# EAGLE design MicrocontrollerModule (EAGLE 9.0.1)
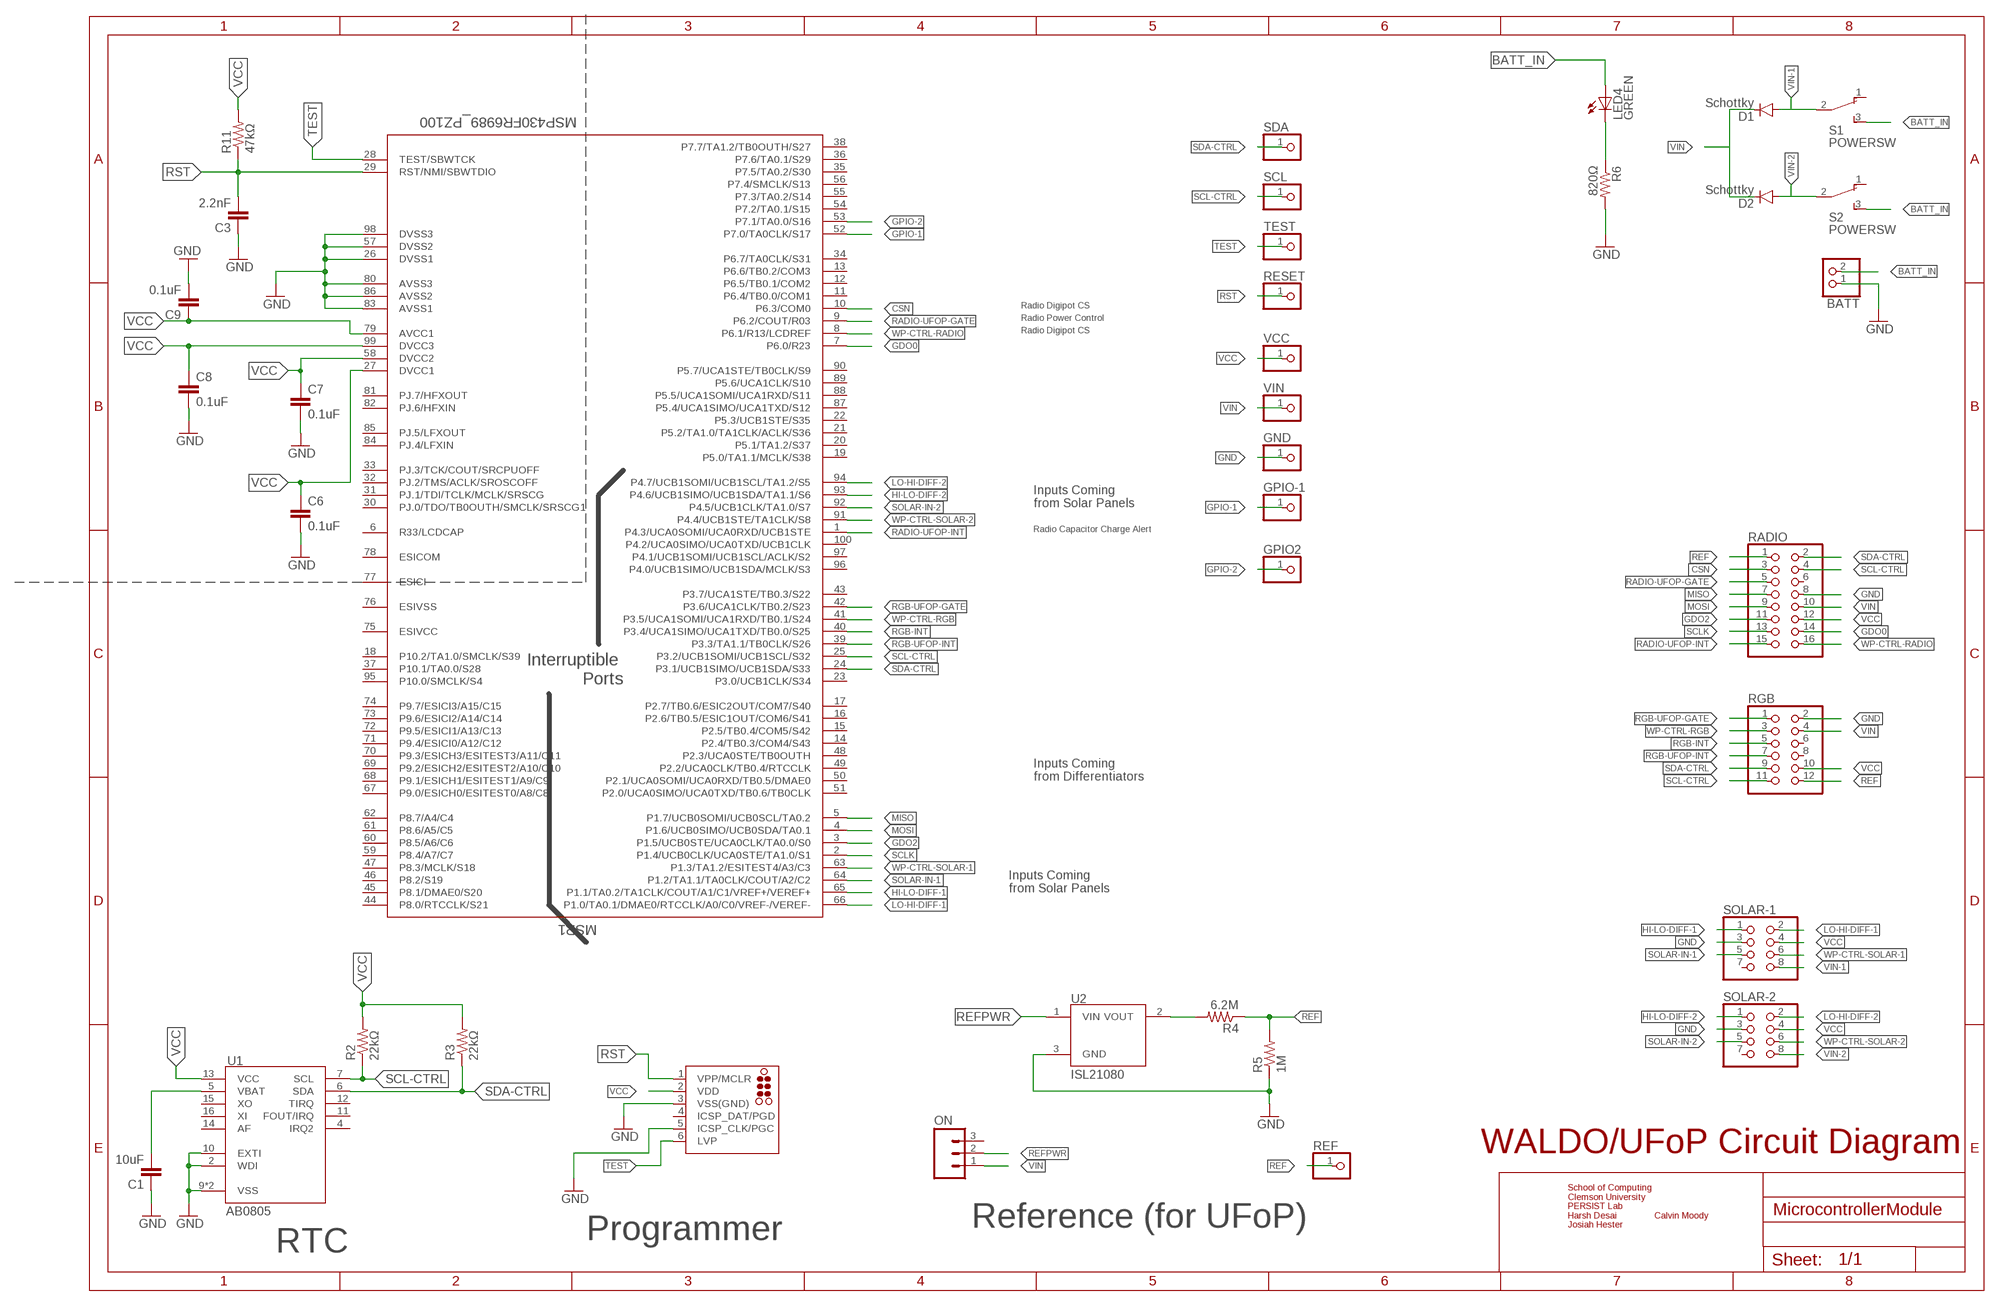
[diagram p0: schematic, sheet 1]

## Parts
BATT  PINHD-1X2  [1X02]
C1  10uF  CAP0805  [0805]
C3  2.2nF  CAP0805  [0805]
C6  0.1uF  CAP0805  [0805]
C7  0.1uF  CAP0805  [0805]
C8  0.1uF  CAP0805  [0805]
C9  0.1uF  CAP0805  [0805]
D1  Schottky  DIODESOD523  [SOD523]
D2  Schottky  DIODESOD523  [SOD523]
GND  PINHD-1X1  [1X01]
GPIO2  PINHD-1X1  [1X01]
GPIO-1  PINHD-1X1  [1X01]
J1  TC2030-MCP-NL  [TC2030-MCP-NL]
LED4  GREEN  LEDCHIP-LED0805  [CHIP-LED0805]
MSP1  MSP430FR6989_PZ100  [PZ100]
ON  M03  [1X03-1.27MM]
R2  22kΩ  RESISTOR0805-RES  [0805]
R3  22kΩ  RESISTOR0805-RES  [0805]
R4  6.2M  RESISTOR0805-RES  [0805]
R5  1M  RESISTOR0805-RES  [0805]
R6  820Ω  RESISTOR0805-RES  [0805]
R11  47kΩ  RESISTOR0805-RES  [0805]
RADIO  PINHD-2X8/90  [2X08/90]
REF  PINHD-1X1  [1X01]
RESET  PINHD-1X1  [1X01]
RGB  PINHD-2X6/90  [2X06/90]
S1  POWERSW  [TL3XYO]
S2  POWERSW  [TL3XYO]
SCL  PINHD-1X1  [1X01]
SDA  PINHD-1X1  [1X01]
SOLAR-1  PINHD-2X4/90  [2X04/90]
SOLAR-2  PINHD-2X4/90  [2X04/90]
TEST  PINHD-1X1  [1X01]
U1  AB0805  [QFN16]
U2  ISL21080  [SOT-23]
VCC  PINHD-1X1  [1X01]
VIN  PINHD-1X1  [1X01]

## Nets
BATT_IN: BATT.2 LED4.A S1.3(S) S2.3(S)
CSN: MSP1.10(P6.3/COM0) RADIO.3
GDO0: MSP1.7(P6.0/R23) RADIO.14
GDO2: MSP1.3(P1.5/UCB0STE/UCA0CLK/TA0.0/S0) RADIO.11
GND: BATT.1 C1.1 C3.1 C6.2 C7.2 C8.2 C9.2 GND.1 J1.3(VSS(GND)) J1.5(ICSP_CLK/PGC) MSP1.26(DVSS1) MSP1.57(DVSS2) MSP1.80(AVSS3) MSP1.83(AVSS1) MSP1.86(AVSS2) MSP1.98(DVSS3) R5.1 R6.2 RADIO.8 RGB.2 SOLAR-1.3 SOLAR-2.3 U1.2(WDI) U1.9(VSS) U1.10(EXTI) U1.TH(VSS) U2.3(GND)
GPIO-1: GPIO-1.1 MSP1.52(P7.0/TA0CLK/S17)
GPIO-2: GPIO2.1 MSP1.53(P7.1/TA0.0/S16)
HI-LO-DIFF-1: MSP1.65(P1.1/TA0.2/TA1CLK/COUT/A1/C1/VREF+/VEREF+) SOLAR-1.1
HI-LO-DIFF-2: MSP1.93(P4.6/UCB1SIMO/UCB1SDA/TA1.1/S6) SOLAR-2.1
LO-HI-DIFF-1: MSP1.66(P1.0/TA0.1/DMAE0/RTCCLK/A0/C0/VREF-/VEREF-) SOLAR-1.2
LO-HI-DIFF-2: MSP1.94(P4.7/UCB1SOMI/UCB1SCL/TA1.2/S5) SOLAR-2.2
MISO: MSP1.5(P1.7/UCB0SOMI/UCB0SCL/TA0.2) RADIO.7
MOSI: MSP1.4(P1.6/UCB0SIMO/UCB0SDA/TA0.1) RADIO.9
N$4: C1.2 U1.5(VBAT)
N$11: LED4.C R6.1
N$12: R4.2 U2.2(VOUT)
RADIO-UFOP-GATE: MSP1.9(P6.2/COUT/R03) RADIO.5
RADIO-UFOP-INT: MSP1.1(P4.3/UCA0SOMI/UCA0RXD/UCB1STE) RADIO.15
REF: R4.1 R5.2 RADIO.1 REF.1 RGB.12
REFPWR: ON.2 U2.1(VIN)
RGB-INT: MSP1.40(P3.4/UCA1SIMO/UCA1TXD/TB0.0/S25) RGB.5
RGB-UFOP-GATE: MSP1.42(P3.6/UCA1CLK/TB0.2/S23) RGB.1
RGB-UFOP-INT: MSP1.39(P3.3/TA1.1/TB0CLK/S26) RGB.7
RST: C3.2 J1.1(VPP/MCLR) MSP1.29(RST/NMI/SBWTDIO) R11.1 RESET.1
SCL-CTRL: MSP1.25(P3.2/UCB1SOMI/UCB1SCL/S32) R2.1 RADIO.4 RGB.11 SCL.1 U1.7(SCL)
SCLK: MSP1.2(P1.4/UCB0CLK/UCA0STE/TA1.0/S1) RADIO.13
SDA-CTRL: MSP1.24(P3.1/UCB1SIMO/UCB1SDA/S33) R3.1 RADIO.2 RGB.9 SDA.1 U1.6(SDA)
SOLAR-IN-1: MSP1.64(P1.2/TA1.1/TA0CLK/COUT/A2/C2) SOLAR-1.5
SOLAR-IN-2: MSP1.92(P4.5/UCB1CLK/TA1.0/S7) SOLAR-2.5
TEST: J1.6(LVP) MSP1.28(TEST/SBWTCK) TEST.1
VCC: C6.1 C7.1 C8.1 C9.1 J1.2(VDD) MSP1.27(DVCC1) MSP1.58(DVCC2) MSP1.79(AVCC1) MSP1.99(DVCC3) R2.2 R3.2 R11.2 RADIO.12 RGB.10 SOLAR-1.4 SOLAR-2.4 U1.13(VCC) VCC.1
VIN: D1.C D2.C ON.1 RADIO.10 RGB.4 VIN.1
VIN-1: D1.A S1.2(P) SOLAR-1.8
VIN-2: D2.A S2.2(P) SOLAR-2.8
WP-CTRL-RADIO: MSP1.8(P6.1/R13/LCDREF) RADIO.16
WP-CTRL-RGB: MSP1.41(P3.5/UCA1SOMI/UCA1RXD/TB0.1/S24) RGB.3
WP-CTRL-SOLAR-1: MSP1.63(P1.3/TA1.2/ESITEST4/A3/C3) SOLAR-1.6
WP-CTRL-SOLAR-2: MSP1.91(P4.4/UCB1STE/TA1CLK/S8) SOLAR-2.6
Unconnected: J1.4(ICSP_DAT/PGD) MSP1.6(R33/LCDCAP) MSP1.11(P6.4/TB0.0/COM1) MSP1.12(P6.5/TB0.1/COM2) MSP1.13(P6.6/TB0.2/COM3) MSP1.14(P2.4/TB0.3/COM4/S43) MSP1.15(P2.5/TB0.4/COM5/S42) MSP1.16(P2.6/TB0.5/ESIC1OUT/COM6/S41) MSP1.17(P2.7/TB0.6/ESIC2OUT/COM7/S40) MSP1.18(P10.2/TA1.0/SMCLK/S39) MSP1.19(P5.0/TA1.1/MCLK/S38) MSP1.20(P5.1/TA1.2/S37) MSP1.21(P5.2/TA1.0/TA1CLK/ACLK/S36) MSP1.22(P5.3/UCB1STE/S35) MSP1.23(P3.0/UCB1CLK/S34) MSP1.30(PJ.0/TDO/TB0OUTH/SMCLK/SRSCG1) MSP1.31(PJ.1/TDI/TCLK/MCLK/SRSCG) MSP1.32(PJ.2/TMS/ACLK/SROSCOFF) MSP1.33(PJ.3/TCK/COUT/SRCPUOFF) MSP1.34(P6.7/TA0CLK/S31) MSP1.35(P7.5/TA0.2/S30) MSP1.36(P7.6/TA0.1/S29) MSP1.37(P10.1/TA0.0/S28) MSP1.38(P7.7/TA1.2/TB0OUTH/S27) MSP1.43(P3.7/UCA1STE/TB0.3/S22) MSP1.44(P8.0/RTCCLK/S21) MSP1.45(P8.1/DMAE0/S20) MSP1.46(P8.2/S19) MSP1.47(P8.3/MCLK/S18) MSP1.48(P2.3/UCA0STE/TB0OUTH) MSP1.49(P2.2/UCA0CLK/TB0.4/RTCCLK) MSP1.50(P2.1/UCA0SOMI/UCA0RXD/TB0.5/DMAE0) MSP1.51(P2.0/UCA0SIMO/UCA0TXD/TB0.6/TB0CLK) MSP1.54(P7.2/TA0.1/S15) MSP1.55(P7.3/TA0.2/S14) MSP1.56(P7.4/SMCLK/S13) MSP1.59(P8.4/A7/C7) MSP1.60(P8.5/A6/C6) MSP1.61(P8.6/A5/C5) MSP1.62(P8.7/A4/C4) MSP1.67(P9.0/ESICH0/ESITEST0/A8/C8) MSP1.68(P9.1/ESICH1/ESITEST1/A9/C9) MSP1.69(P9.2/ESICH2/ESITEST2/A10/C10) MSP1.70(P9.3/ESICH3/ESITEST3/A11/C11) MSP1.71(P9.4/ESICI0/A12/C12) MSP1.72(P9.5/ESICI1/A13/C13) MSP1.73(P9.6/ESICI2/A14/C14) MSP1.74(P9.7/ESICI3/A15/C15) MSP1.75(ESIVCC) MSP1.76(ESIVSS) MSP1.77(ESICI) MSP1.78(ESICOM) MSP1.81(PJ.7/HFXOUT) MSP1.82(PJ.6/HFXIN) MSP1.84(PJ.4/LFXIN) MSP1.85(PJ.5/LFXOUT) MSP1.87(P5.4/UCA1SIMO/UCA1TXD/S12) MSP1.88(P5.5/UCA1SOMI/UCA1RXD/S11) MSP1.89(P5.6/UCA1CLK/S10) MSP1.90(P5.7/UCA1STE/TB0CLK/S9) MSP1.95(P10.0/SMCLK/S4) MSP1.96(P4.0/UCB1SIMO/UCB1SDA/MCLK/S3) MSP1.97(P4.1/UCB1SOMI/UCB1SCL/ACLK/S2) MSP1.100(P4.2/UCA0SIMO/UCA0TXD/UCB1CLK) ON.3 RADIO.6 RGB.6 RGB.8 S1.1(O) S2.1(O) SOLAR-1.7 SOLAR-2.7 U1.4(IRQ2) U1.11(FOUT/IRQ) U1.12(TIRQ) U1.14(AF) U1.15(XO) U1.16(XI)

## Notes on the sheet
- Radio Digipot CS
- Radio Power Control
- Radio Digipot CS
- Inputs Coming 
  from Solar Panels
- Radio Capacitor Charge Alert
- Interruptible 
  Ports
- Inputs Coming 
  from Differentiators
- Inputs Coming 
  from Solar Panels
- WALDO/UFoP Circuit Diagram
- Reference (for UFoP)
- School of Computing
  Clemson University
  PERSIST Lab
  Harsh Desai               Calvin Moody
  Josiah Hester
- Programmer
- RTC

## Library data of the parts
BATT = pinhead:PINHD-1X2: PIN HEADER
C1 C3 C6-C9 = SparkFun-Capacitors:CAP: Capacitor
D1 D2 = SparkFun-DiscreteSemi:DIODE: Diode
GND GPIO2 GPIO-1 REF RESET SCL SDA TEST VCC VIN = adafruit:PINHD-1X1: Pin header 1x1 for 0.1" spacing
J1 = tag-connect_msp430:TC2030: TAG-CONNECT ICSP Connector Manufacturer: Tag-Connect Cable for easy In-Circuit Serial Programming. Designed for Microchip ICD2, suitable for many others. Two variants - one "with legs" (for hands-free fit on PCB) and another "without legs" for quick programming. PADDescription 1MCLR/Vpp 2Vdd 3GND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
LED4 = led:LED: LED
MSP1 = msp430:MSP430FR6989_PZ100
ON = SparkFun-Connectors:M03: Header 3 Standard 3-pin 0.1" header. Use with straight break away headers (SKU : PRT-00116), right angle break away headers (PRT-00553), swiss pins (PRT-00743), machine pins (PRT-00117), and female headers (PRT-00115). Molex polarized connector foot print use with SKU : PRT-08232 with associated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
R2 R3 R6 R11 = SparkFun-Resistors:RESISTOR: Resistor
R4 = SparkFun-Resistors:RESISTOR: Resistor; DIGIKEY: 541-6.20MHCT-ND
R5 = SparkFun-Resistors:RESISTOR: Resistor; DIGIKEY: 311-1.00MHRCT-ND
RADIO = pinhead:PINHD-2X8: PIN HEADER
RGB = pinhead:PINHD-2X6: PIN HEADER
S1 S2 = GreenBoard:POWERSW: TINY SWITCH ON - ON Source: http://www2.produktinfo.conrad.com/datenblaetter/700000-724999/705152-da-01-de-Subminiaturschalter_TL_36YO.pdf
SOLAR-1 SOLAR-2 = pinhead:PINHD-2X4: PIN HEADER
U1 = AB08XX:AB0805: AB08X5 Real-Time Clock Family: I2C Version The ABRACON AB08X5 Real-Time Clock family provides a groundbreaking combination of ultra-low power coupled with a highly sophisticated feature set. With power requirements significantly lower than any other industry RTC (as low as 14 nA), these are the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; MOUSER: 815-AB0805-T3
U2 = isl21080:ISL21080: Intersil: ISL21080, 300nA NanoPower Voltage References The ISL21080 analog voltage references feature low supply voltage operation at ultra-low 310nA typ, 1.5µA max operating current. Additionally, the ISL21080 family features guaranteed initial accuracy as low as ±0.2% and 50ppm/°C temperature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; DIGIKEY: ISL21080DIH309Z-TKCT-ND

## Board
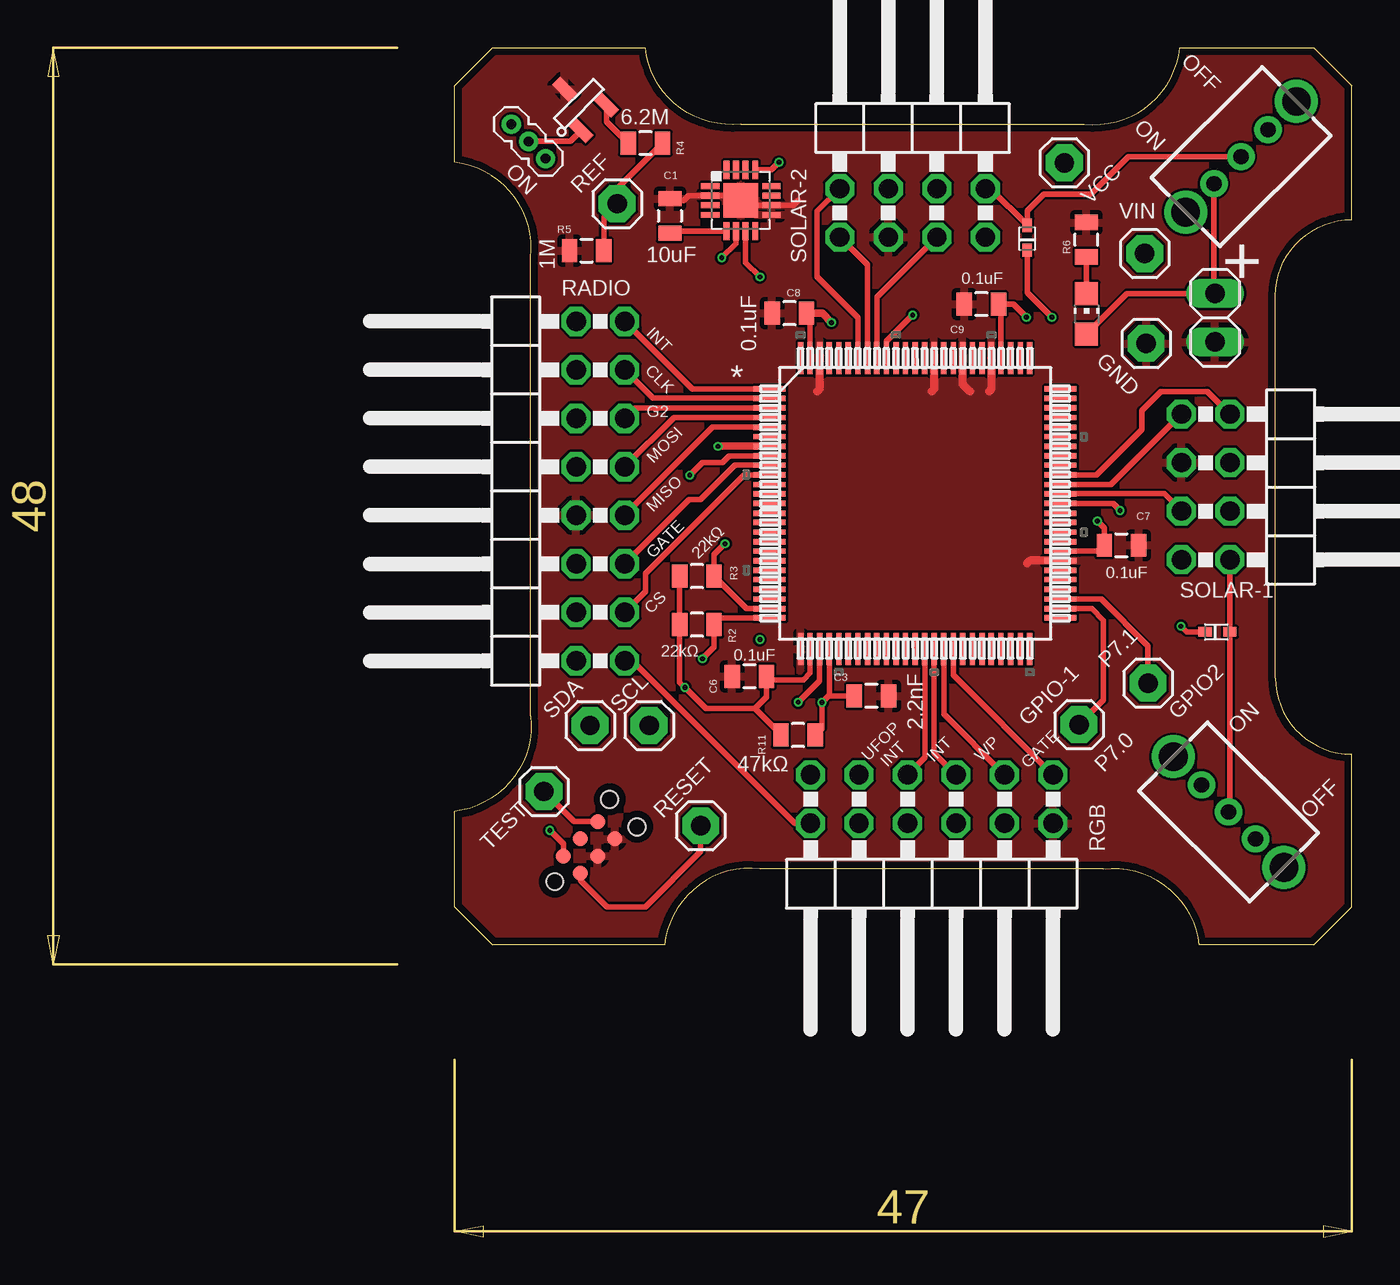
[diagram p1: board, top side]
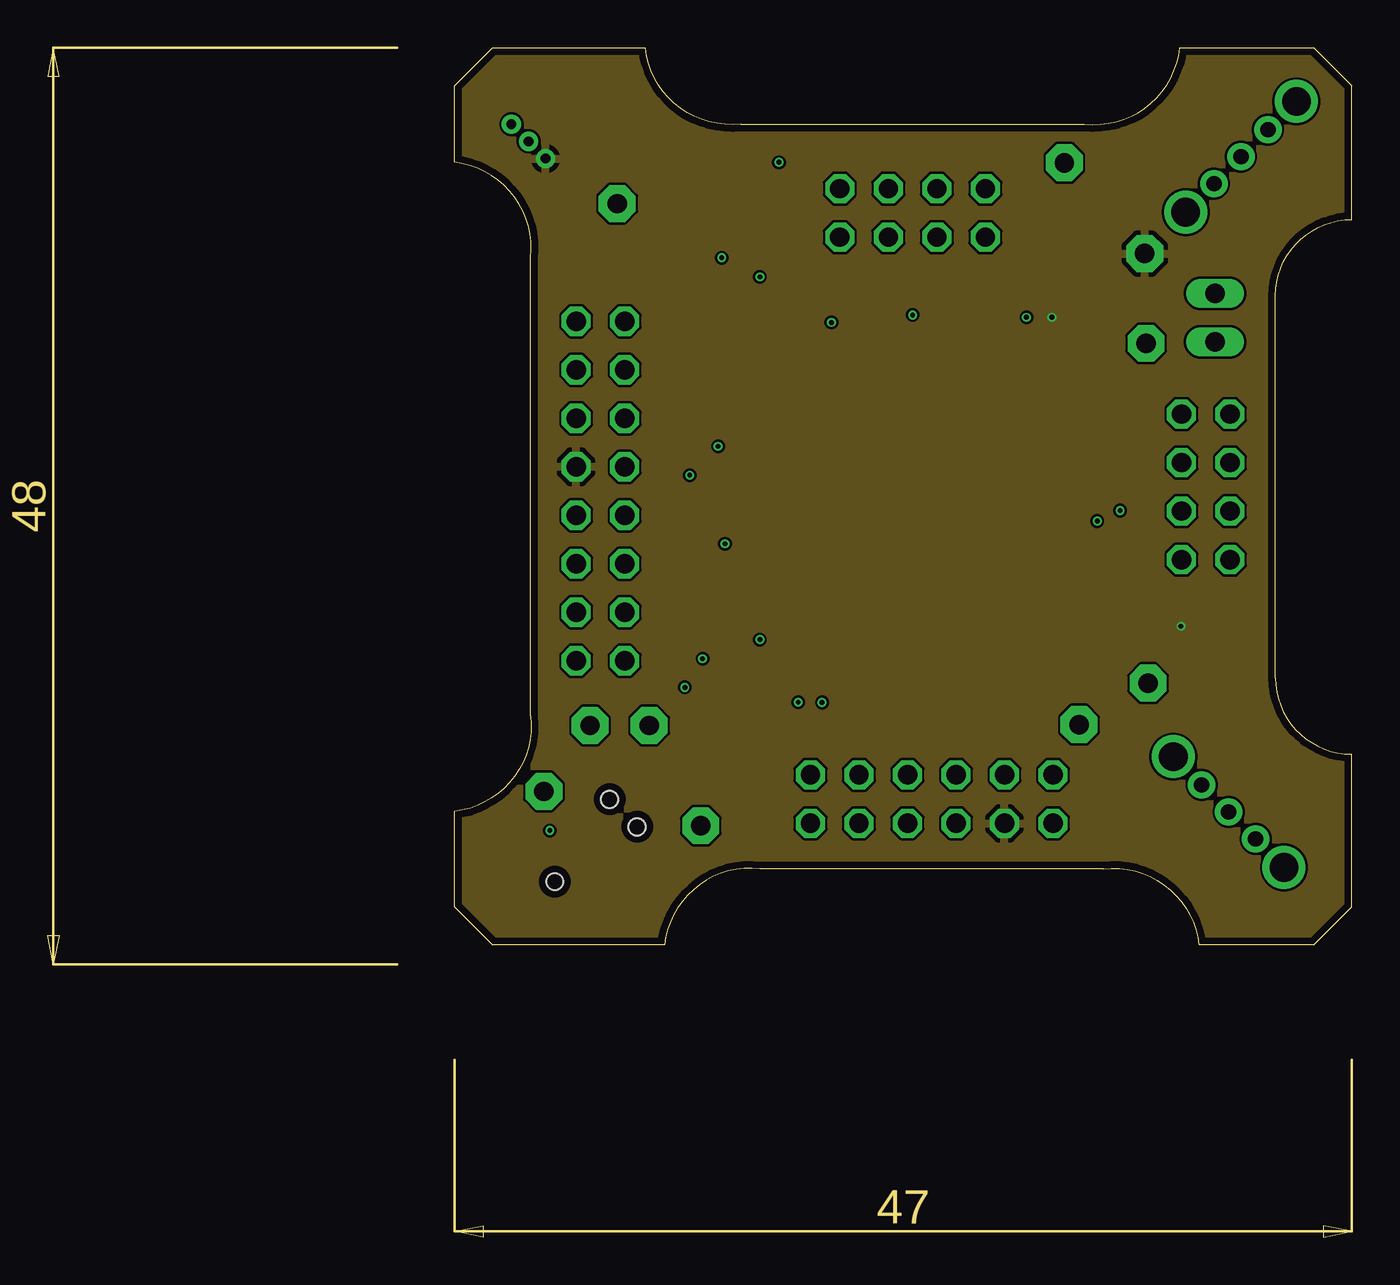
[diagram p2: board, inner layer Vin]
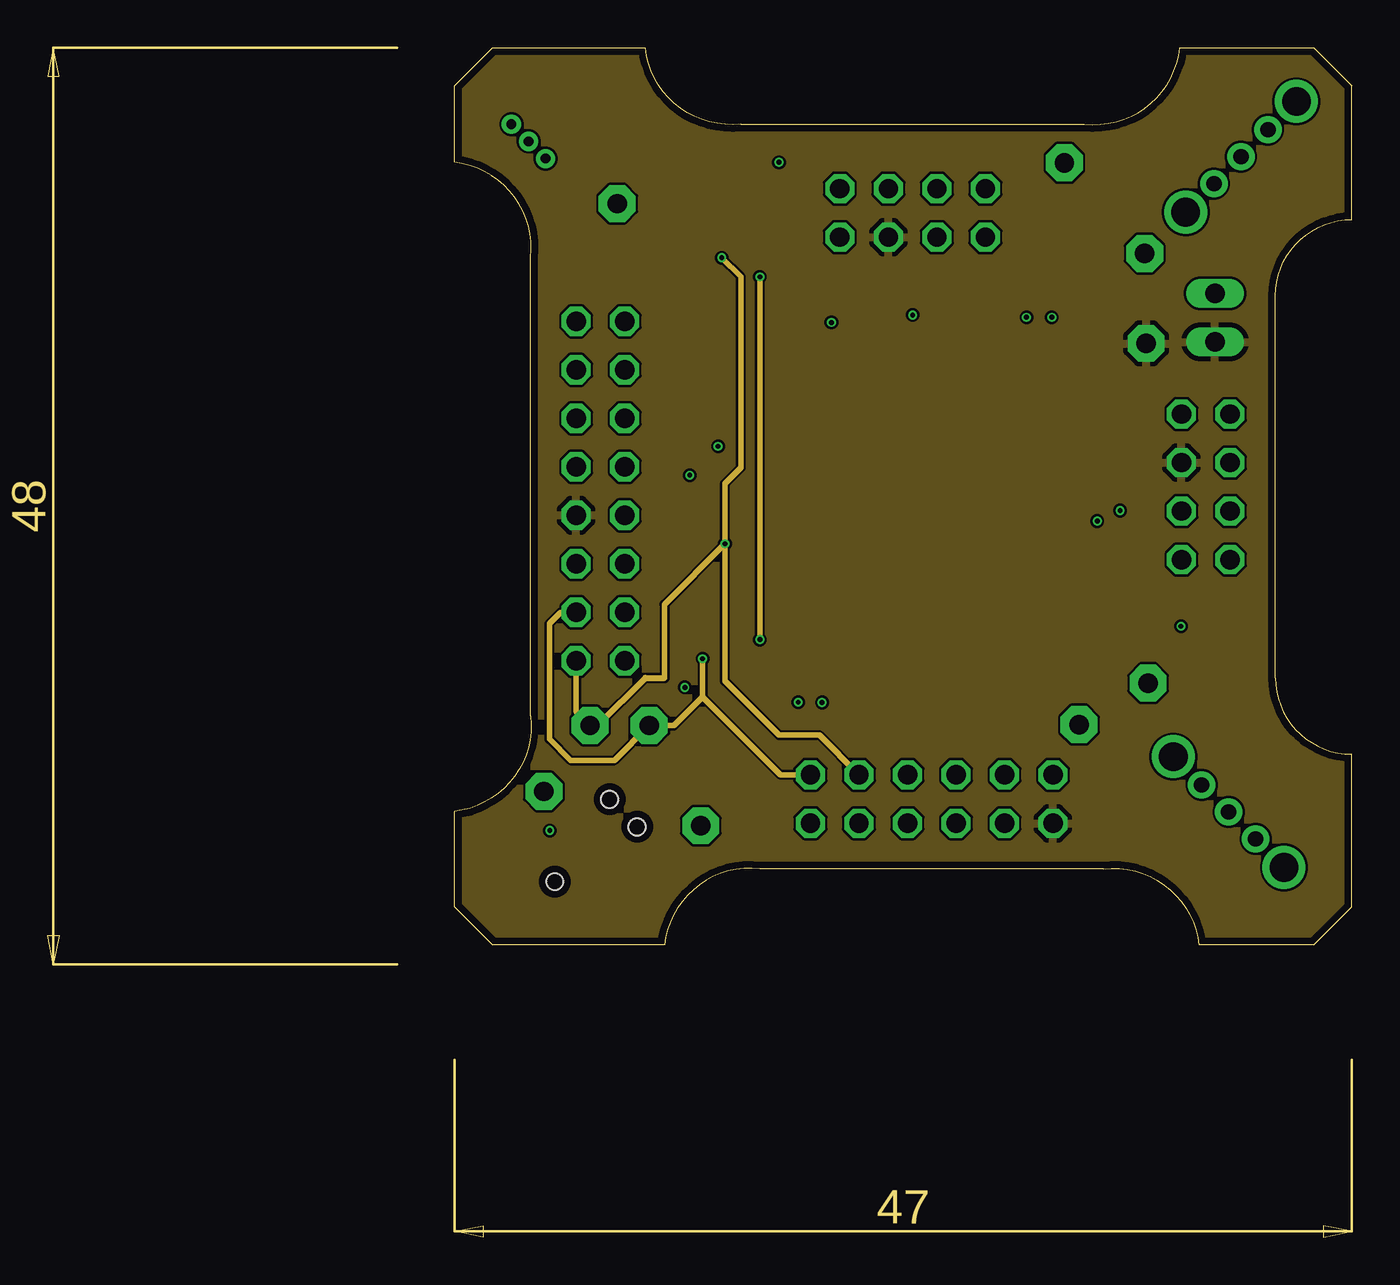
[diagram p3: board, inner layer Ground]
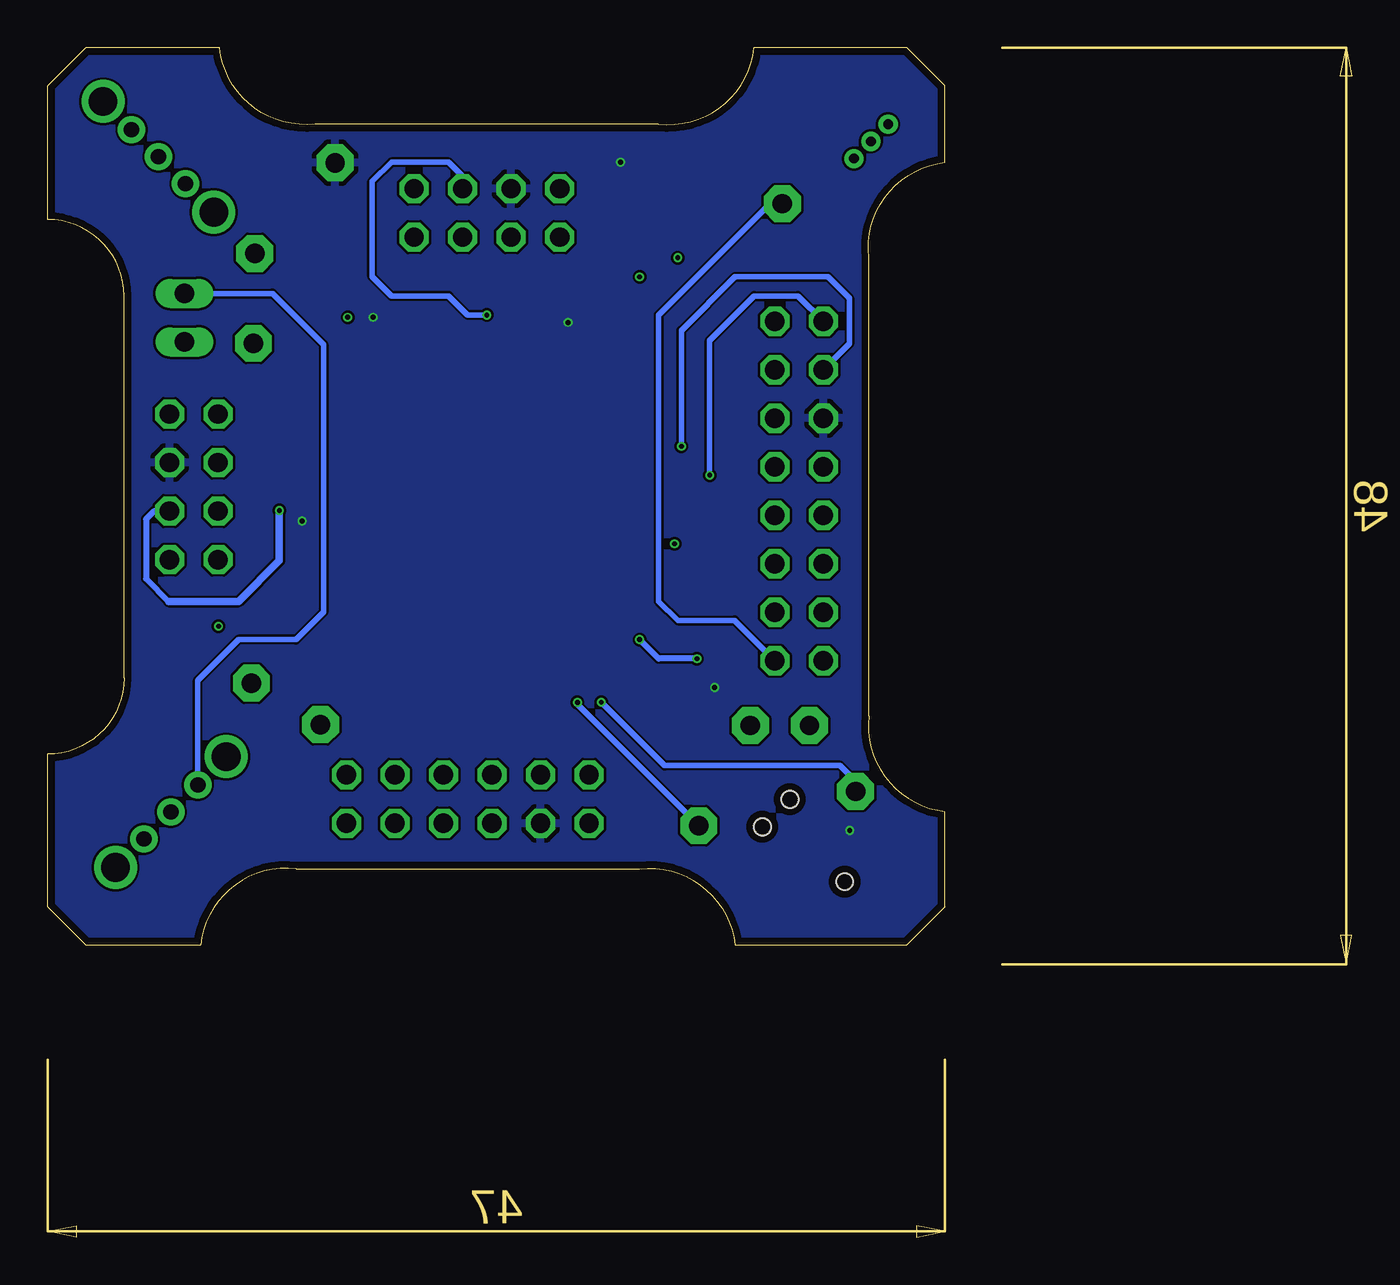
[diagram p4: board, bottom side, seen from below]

Size 68.3 x 62.3 mm. Coordinates in mm from the lower left corner, seen from the top.
Outline: 36.3,58.3 54.3,58.3 arc90 59.3,62.3 66.3,62.3 68.3,60.3 68.3,53.3 arc90 64.3,49.3 64.3,29.3 arc90 68.3,25.3 68.3,17.3 66.3,15.3 60.3,15.3 arc90 55.3,19.3 37.3,19.3 arc90 32.3,15.3 23.3,15.3 21.3,17.3 21.3,22.3 arc90 25.3,27.3 25.3,51.3 arc90 21.3,56.3 21.3,60.3 23.3,62.3 31.3,62.3 arc90 36.3,58.3
Copper layers (1*2*15*16): Top 0.035559375mm / dielectric 0.17018125mm / Vin 0.01778125mm / dielectric 47mil / Ground 0.01778125mm / dielectric 0.17018125mm / Bottom 0.035559375mm
Design rules "OSHPark-4layer": minimum track width 5mil, minimum drill 10mil, track to track 5mil, track to pad 5mil, pad to pad 5mil, via to via 5mil, smd to smd 5mil, copper to edge 15mil, drill to drill 6mil, minimum pad ring 4mil, minimum via ring 4mil, stop-mask expansion 2.5mil, vias tented up to drill 0mil, thermal gap 10mil

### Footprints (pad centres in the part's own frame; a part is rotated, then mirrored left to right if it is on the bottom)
1X02 = drill 1.016 long: 1 -1.27,0; 2 1.27,0
0805 = smd 0.8 x 1.2: 1 -0.9,0; 2 0.9,0
SOD523 = smd 0.7 x 0.5: A 0.7,0; C -0.6,0
1X01 = drill 1.016 pad 1.93 octagon: 1 0,0
TC2030-MCP-NL = smd 0.787 x 0.787: 1 1.27,-0.635; 2 1.27,0.635; 3 2.54,-0.635; 4 2.54,0.635; 5 3.81,-0.635; 6 3.81,0.635 | hole 0.889: 0,0; 5.08,-1.016; 5.08,1.016
CHIP-LED0805 = smd 1.2 x 1.2: A 0,-1.05; C 0,1.05
PZ100 = smd 1.676 x 0.279: 1 -7.62,5.994; 2 -7.62,5.512; 3 -7.62,5.004; 4 -7.62,4.496; 5 -7.62,3.988; 6 -7.62,3.505; 7 -7.62,2.997; 8 -7.62,2.489; 9 -7.62,2.007; 10 -7.62,1.499; 11 -7.62,0.991; 12 -7.62,0.508; 13 -7.62,0; 14 -7.62,-0.508; 15 -7.62,-0.991; 16 -7.62,-1.499; 17 -7.62,-2.007; 18 -7.62,-2.489; 19 -7.62,-2.997; 20 -7.62,-3.505; 21 -7.62,-3.988; 22 -7.62,-4.496; 23 -7.62,-5.004; 24 -7.62,-5.512; 25 -7.62,-5.994; 51 7.62,-5.994; 52 7.62,-5.512; 53 7.62,-5.004; 54 7.62,-4.496; 55 7.62,-3.988; 56 7.62,-3.505; 57 7.62,-2.997; 58 7.62,-2.489; 59 7.62,-2.007; 60 7.62,-1.499; 61 7.62,-0.991; 62 7.62,-0.508; 63 7.62,0; 64 7.62,0.508; 65 7.62,0.991; 66 7.62,1.499; 67 7.62,2.007; 68 7.62,2.489; 69 7.62,2.997; 70 7.62,3.505; 71 7.62,3.988; 72 7.62,4.496; 73 7.62,5.004; 74 7.62,5.512; 75 7.62,5.994 | smd 0.279 x 1.676: 26 -5.994,-7.62; 27 -5.512,-7.62; 28 -5.004,-7.62; 29 -4.496,-7.62; 30 -3.988,-7.62; 31 -3.505,-7.62; 32 -2.997,-7.62; 33 -2.489,-7.62; 34 -2.007,-7.62; 35 -1.499,-7.62; 36 -0.991,-7.62; 37 -0.508,-7.62; 38 0,-7.62; 39 0.508,-7.62; 40 0.991,-7.62; 41 1.499,-7.62; 42 2.007,-7.62; 43 2.489,-7.62; 44 2.997,-7.62; 45 3.505,-7.62; 46 3.988,-7.62; 47 4.496,-7.62; 48 5.004,-7.62; 49 5.512,-7.62; 50 5.994,-7.62; 76 5.994,7.62; 77 5.512,7.62; 78 5.004,7.62; 79 4.496,7.62; 80 3.988,7.62; 81 3.505,7.62; 82 2.997,7.62; 83 2.489,7.62; 84 2.007,7.62; 85 1.499,7.62; 86 0.991,7.62; 87 0.508,7.62; 88 0,7.62; 89 -0.508,7.62; 90 -0.991,7.62; 91 -1.499,7.62; 92 -2.007,7.62; 93 -2.489,7.62; 94 -2.997,7.62; 95 -3.505,7.62; 96 -3.988,7.62; 97 -4.496,7.62; 98 -5.004,7.62; 99 -5.512,7.62; 100 -5.994,7.62
1X03-1.27MM = drill 0.508 pad 1: 1 -1.27,0; 2 0,0; 3 1.27,0
2X08/90 = drill 1.016 octagon: 1 -8.89,-6.35; 2 -8.89,-3.81; 3 -6.35,-6.35; 4 -6.35,-3.81; 5 -3.81,-6.35; 6 -3.81,-3.81; 7 -1.27,-6.35; 8 -1.27,-3.81; 9 1.27,-6.35; 10 1.27,-3.81; 11 3.81,-6.35; 12 3.81,-3.81; 13 6.35,-6.35; 14 6.35,-3.81; 15 8.89,-6.35; 16 8.89,-3.81
2X06/90 = drill 1.016 octagon: 1 -6.35,-6.35; 2 -6.35,-3.81; 3 -3.81,-6.35; 4 -3.81,-3.81; 5 -1.27,-6.35; 6 -1.27,-3.81; 7 1.27,-6.35; 8 1.27,-3.81; 9 3.81,-6.35; 10 3.81,-3.81; 11 6.35,-6.35; 12 6.35,-3.81
TL3XYO = drill 0.8 pad 1.422: 1 -2,0; 2 0,0; 3 2,0 | drill 1.5 pad 1.93: M1 -4.1,0; M2 4.1,0
2X04/90 = drill 1.016 octagon: 1 -3.81,-6.35; 2 -3.81,-3.81; 3 -1.27,-6.35; 4 -1.27,-3.81; 5 1.27,-6.35; 6 1.27,-3.81; 7 3.81,-6.35; 8 3.81,-3.81
QFN16 = smd 0.95 x 0.3: 1 -1.6,0.75; 2 -1.6,0.25; 3 -1.6,-0.25; 4 -1.6,-0.75; 9 1.6,-0.75; 10 1.6,-0.25; 11 1.6,0.25; 12 1.6,0.75 | smd 0.3 x 0.95: 5 -0.75,-1.6; 6 -0.25,-1.6; 7 0.25,-1.6; 8 0.75,-1.6; 13 0.75,1.6; 14 0.25,1.6; 15 -0.25,1.6; 16 -0.75,1.6 | smd 1.8 x 1.8: TH 0,0
SOT-23 = smd 0.6 x 1.25: 1 -0.95,-1.075; 2 0.95,-1.075; 3 -0.025,1.075

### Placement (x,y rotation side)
BATT  61.14,48.16 90 top
C1  32.59,53.49 270 top
C3  43.14,28.35 180 top
C6  36.75,29.37 180 top
C7  56.24,36.24 0 top
C8  38.84,48.39 180 top
C9  48.9,48.87 180 top
D1  [SOD523]  61.21,31.7 0 top
D2  [SOD523]  51.3,52.3 90 top
GND  57.53,46.81 0 top
GPIO2  57.63,29.02 0 top
GPIO-1  54.02,26.85 0 top
J1  26.56,18.62 45 top
LED4  54.41,48.36 0 top
MSP1  45.43,38.43 0 top
ON  25.18,57.39 135 top
R2  34,32.08 180 top
R3  34,34.62 180 top
R4  31.3,57.3 180 top
R5  28.23,51.67 0 top
R6  54.4,52.25 90 top
R11  39.3,26.3 180 top
RADIO  23.87,39.08 90 top
REF  29.83,54.13 0 top
RESET  34.2,21.55 0 top
RGB  46.3,17.87 180 top
S1  61.85,22.27 135 top
S2  62.5,56.59 225 top
SCL  31.5,26.8 0 top
SDA  28.41,26.8 0 top
SOLAR-1  65.73,39.3 270 top
SOLAR-2  45.3,58.73 0 top
TEST  25.99,23.34 0 top
U1  36.3,54.3 0 top
U2  27.84,59.38 45 top
VCC  53.25,56.28 0 top
VIN  57.45,51.52 0 top

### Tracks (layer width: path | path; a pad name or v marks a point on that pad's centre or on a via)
BATT_IN
  Top 0.279: S2.3 61.09,49.48 | BATT.2 56.53,49.43 LED4.A
  Top 0.305: 61.09,49.48 BATT.2
  Bottom 0.279: BATT.2 56.53,49.43 53.86,46.76 53.86,32.74 55.3,31.3 58.3,31.3 60.44,29.16 S1.3
CSN
  Top 0.279: MSP1.10 36.47,39.93 31.3,34.76 31.3,33.81 RADIO.3
GDO0  (via drill 0.25)
  Top 0.381: MSP1.7 v35.12,41.43 v35.11,41.42
  Bottom 0.279: v35.11,41.42 35.11,47.49 32.3,50.3 27.43,50.3 26.31,49.18 26.31,46.8 RADIO.14
GDO2
  Top 0.279: MSP1.3 30.76,43.43 RADIO.11
GND
  Top 0.279: 36.05,54.55 U1.2 33.55,54.55 33.3,54.3 | U1.TH 36.55,54.05 U1.10 39.05,54.05
  Top 0.305: U1.TH 36.05,54.55 | 39.05,54.05 39.3,54.3
  Top 0.406: MSP1.86 46.42,44.42 46.3,44.3 | MSP1.83 47.92,44.68 48.3,44.3 | MSP1.80 49.42,44.42 49.3,44.3 | MSP1.98 40.43,44.43 40.3,44.3 | MSP1.57 51.43,35.43 51.3,35.3
  pour Top: 20.03,13.03 20.03,64.02 77.18,64.02 77.18,13.03
  pour Ground: 14.95,67.83 14.95,9.22 80.99,9.22 80.99,67.83
GPIO-1
  Top 0.279: MSP1.52 54.68,32.92 55.3,32.3 55.3,28.13 GPIO-1.1
GPIO-2
  Top 0.279: MSP1.53 55.17,33.43 57.63,30.97 GPIO2.1
HI-LO-DIFF-1
  Top 0.279: MSP1.65 55.69,39.42 SOLAR-1.1
HI-LO-DIFF-2
  Top 0.279: MSP1.93 42.94,50.93 SOLAR-2.1
LO-HI-DIFF-1
  Top 0.279: MSP1.66 54.93,39.93 57.3,42.3 57.3,43.3 58.3,44.3 60.73,44.3 SOLAR-1.2
LO-HI-DIFF-2
  Top 0.279: MSP1.94 42.43,48.17 40.3,50.3 40.3,53.73 SOLAR-2.2
MISO
  Top 0.279: MSP1.5 34.83,42.42 RADIO.7
MOSI
  Top 0.279: MSP1.4 32.8,42.93 RADIO.9
N$4
  Top 0.279: U1.5 32.7,52.7
  Top 0.305: 32.7,52.7 C1.2
N$11
  Top 0.279: R6.1 LED4.C
  Top 0.305: LED4.C
N$12
  Top 0.279: U2.2 29.27,58.43 R4.2
RADIO-UFOP-GATE
  Top 0.279: MSP1.9 35.99,40.44 34.19,38.64 33.59,38.64 RADIO.5
RADIO-UFOP-INT
  Top 0.279: RADIO.15 33.77,44.42 MSP1.1
REF
  Top 0.279: RADIO.1 30.62,30.19 39.13,21.68 RGB.12 | R4.1 29.83,54.93 REF.1 29.13,53.43 R5.2
  Top 0.305: REF.1
  Bottom 0.279: RADIO.1 32.33,32.3 35.3,32.3 36.3,33.3 36.3,48.3 30.47,54.13 REF.1
REFPWR
  Top 0.279: ON.2 27.37,57.39 U2.1
RGB-INT
  Top 0.279: MSP1.40 46.42,25.37 RGB.5
RGB-UFOP-GATE
  Top 0.279: MSP1.42 47.44,29.43 RGB.1
RGB-UFOP-INT
  Top 0.279: MSP1.39 45.94,25.13 RGB.7
RST  (via drill 0.25)
  Top 0.279: J1.1 27.91,18.7 29.3,17.3 31.3,17.3 34.2,20.2 RESET.1 | MSP1.29 40.93,28.39 v40.55,28.01 40.55,26.65 R11.1 | C3.2 40.97,28.35
  Top 0.305: 40.97,28.35 40.93,28.39
  Bottom 0.279: 40.55,27.91 RESET.1
  Bottom 0.305: v40.55,28.01 40.55,27.91
SCL-CTRL  (via drill 0.25)
  Top 0.279: MSP1.25 35.26,32.44 R2.1 34.9,30.9 v34.3,30.3 | U1.7 36.55,51.05 v37.3,50.3
  Ground 0.279: RADIO.4 26.87,32.73 26.28,32.14 26.28,26.09 27.39,24.98 29.68,24.98 SCL.1 32.8,26.8 34.3,28.3 | RGB.11 38.38,24.22 34.3,28.3 | v37.3,31.3 v37.3,50.3 | v34.3,30.3 34.3,28.3
  Bottom 0.305: v34.3,30.3 36.3,30.3 v37.3,31.3
SCLK
  Top 0.279: MSP1.2 31.71,43.94 RADIO.13
SDA-CTRL  (via drill 0.25)
  Top 0.279: MSP1.24 36.6,32.92 R3.1 34.9,35.75 v35.47,36.32 | U1.6 36.05,52.05 v35.3,51.3
  Ground 0.279: 32.3,29.3 32.3,33.15 v35.47,36.32 | RGB.9 40.41,26.3 38.3,26.3 35.47,29.13 v35.47,36.32 | v35.47,36.32 35.47,39.47 36.3,40.3 36.3,50.3 v35.3,51.3 | RADIO.2 27.68,27.53 SDA.1 28.8,26.8 31.3,29.3
  Ground 0.305: 31.3,29.3 32.3,29.3
SOLAR-IN-1
  Top 0.279: MSP1.64 58.47,38.94 SOLAR-1.5
SOLAR-IN-2
  Top 0.279: SOLAR-2.5 43.42,49.23 MSP1.92
TEST  (via drill 0.25)
  Top 0.279: MSP1.28 40.43,29.14 v39.3,28.02 | J1.6 27.57,21.76 TEST.1
  Bottom 0.279: TEST.1 25.99,23.88 26.81,24.7 35.99,24.7 v39.3,28.02
VCC  (via drill 0.25)
  Top 0.279: MSP1.79 49.93,48.74 | MSP1.99 39.92,48.21 | MSP1.58 55.04,35.94 C7.1 55.34,37.14 v54.97,37.51 | MSP1.27 39.92,29.54 39.57,29.19 37.83,29.19 C6.1 37.65,28.29 37.04,27.68 | C9.1 50.59,48.87 v51.26,48.18 | R3.2 R2.2 33.1,29.07 v33.37,28.8 34.49,27.68 34.64,27.68 37.04,27.68 | J1.2 27.01,20.59 v26.3,21.3 | U1.13 37.9,55.9 v38.3,56.3 | 38.4,26.32 37.04,27.68
  Top 0.305: R11.2 38.4,26.32
  Top 0.381: 37.72,29.3 C6.1 | C8.1 40.57,48.39 v41.05,47.91
  Top 0.406: 49.93,48.74 C9.1 | 39.92,48.21 C8.1
  pour Bottom: 17.49,11.76 17.49,65.29 70.83,65.29 78.45,53.67 78.45,11.76
VIN  (via drill 0.25)
  Top 0.279: v52.59,48.18 51.3,49.47 D2.C | D1.C 59.65,31.7 v59.36,32
  pour Vin: 16.22,67.56 16.22,10.49 79.72,10.49 79.72,67.56
VIN-1
  Top 0.279: SOLAR-1.8 D1.A | D1.A 61.91,22.33 S1.2
  Top 0.305: D1.A
VIN-2
  Top 0.279: 49.38,54.92 D2.A 51.3,53.77 52.17,54.64 54.64,54.64 56.59,56.59 S2.2
  Top 0.406: SOLAR-2.8 49.38,54.92
WP-CTRL-RADIO  (via drill 0.25)
  Top 0.279: MSP1.8 35.68,40.92 35.34,40.58 34.3,40.58 v33.63,39.91
  Bottom 0.279: v33.63,39.91 33.63,46.97 31.3,49.3 29.01,49.3 RADIO.16
WP-CTRL-RGB
  Top 0.279: MSP1.41 46.93,27.4 RGB.3
WP-CTRL-SOLAR-1  (via drill 0.25)
  Top 0.279: MSP1.63 55.8,38.43 v56.17,38.06
  Bottom 0.305: SOLAR-1.6 62.73,38.03 63.15,37.61 63.15,34.49 61.96,33.3
  Bottom 0.381: v56.17,38.06 56.17,35.43 58.3,33.3 61.96,33.3
WP-CTRL-SOLAR-2  (via drill 0.25)
  Top 0.279: MSP1.91 43.93,46.93 v45.3,48.3
  Bottom 0.279: v45.3,48.3 46.3,48.3 47.3,49.3 50.3,49.3 51.3,50.3 51.3,55.3 50.3,56.3 47.3,56.3 46.57,55.57 | 46.57,55.57 SOLAR-2.6 46.57,55.57

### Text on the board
tPlace: OFF | ON | + | INT | CLK | G2 | MOSI | MISO | GATE | CS | P7.1 | ON | UFOP / INT | INT | WP | GATE | P7.0 | OFF

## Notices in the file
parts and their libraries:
SparkFun-Capacitors: Licensing: Creative Commons ShareAlike 4.0 International - https://creativecommons.org/licenses/by-sa/4.0
tag-connect_msp430: ©2009 ROFA.cz - modified and updated by Robert Darlington ‹rdarlington@gmail.com›
